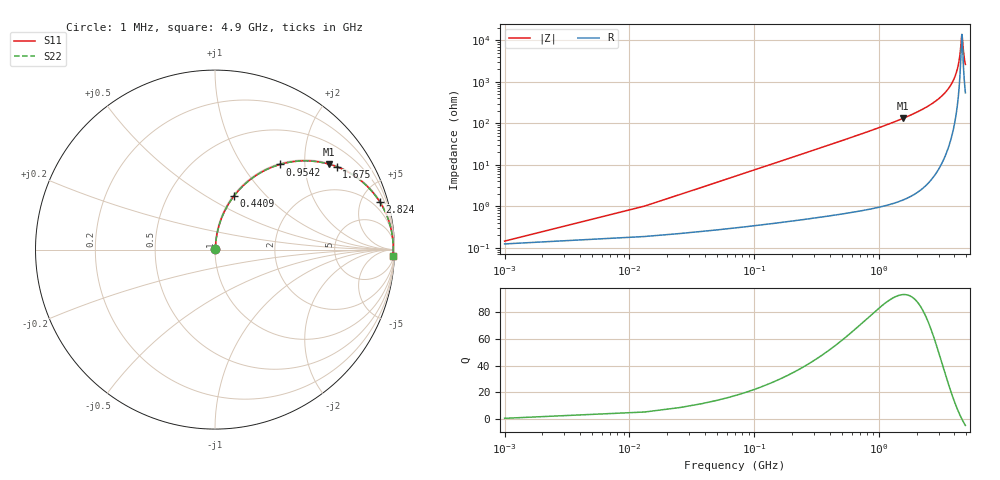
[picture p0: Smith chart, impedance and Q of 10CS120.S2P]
! Coilcraft 1008CS-120 Chip Inductor
! 02 July 2002
# MHZ S MA R 50
!Freq  MagS11  AngS11  MagS21  AngS21  MagS12  AngS12  MagS22  AngS22
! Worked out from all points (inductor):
!   402 points, 1 MHz to 4.9 GHz, reference 50 ohm
!   read as one part in series: L = 12 nH near 25.44 MHz
!   highest Q = 93 at 1.553 GHz (marker M1), where L = 13.5 nH
!   self-resonance near 4.583 GHz
!   S11 on the Smith chart (normalised r, x): 1 MHz: 1.00, +0.00; 440.9 MHz: 1.01, +0.67; 954.2 MHz: 1.02, +1.50; 1.675 GHz: 1.03, +2.91; 2.824 GHz: 1.12, +6.84; 4.9 GHz: 12, -52
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1  0.001449 31.3  0.9988 -0.0  0.9988 -0.0  0.001449 31.3
37.66  0.02842 83.4  0.9971 -1.6  0.9971 -1.6  0.02842 83.4
62.1  0.04673 83.8  0.996 -2.7  0.996 -2.7  0.04673 83.8
98.76  0.07412 83.2  0.9939 -4.2  0.9939 -4.2  0.07412 83.2
159.86  0.1194 81.2  0.9889 -6.9  0.9889 -6.9  0.1194 81.2
233.18  0.1729 78.5  0.9804 -10.0  0.9804 -10.0  0.1729 78.5
440.92  0.3164 70.5  0.9429 -18.4  0.9429 -18.4  0.3164 70.5
819.74  0.5349 56.9  0.8379 -32.3  0.8379 -32.3  0.5349 56.9
954.16  0.5975 52.6  0.7946 -36.7  0.7946 -36.7  0.5975 52.6
1552.94  0.7934 36.9  0.6002 -52.5  0.6002 -52.5  0.7934 36.9
1638.48  0.8126 35.0  0.5741 -54.3  0.5741 -54.3  0.8126 35.0
1675.14  0.8203 34.3  0.5631 -55.1  0.5631 -55.1  0.8203 34.3
2457.22  0.9288 21.0  0.358 -68.2  0.358 -68.2  0.9288 21.0
2823.82  0.9554 16.2  0.2793 -72.8  0.2793 -72.8  0.9554 16.2
3275.96  0.9758 11.2  0.1943 -77.3  0.1943 -77.3  0.9758 11.2
3752.54  0.9876 6.7  0.1164 -80.5  0.1164 -80.5  0.9876 6.7
4094.7  0.9916 3.8  0.06643 -80.9  0.06643 -80.9  0.9916 3.8
4375.76  0.9929 1.6  0.02885 -75.0  0.02885 -75.0  0.9929 1.6
4559.06  0.9929 0.3  0.008394 -32.4  0.008394 -32.4  0.9929 0.3
4595.72  0.9929 -0.0  0.007138 0.4  0.007138 0.4  0.9929 -0.0
4766.8  0.9923 -1.2  0.02228 69.1  0.02228 69.1  0.9923 -1.2
4900  0.9915 -2.1  0.03757 75.9  0.03757 75.9  0.9915 -2.1
